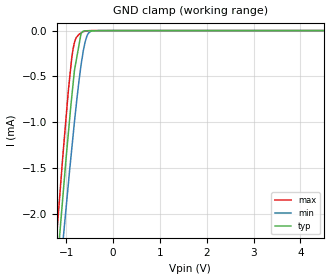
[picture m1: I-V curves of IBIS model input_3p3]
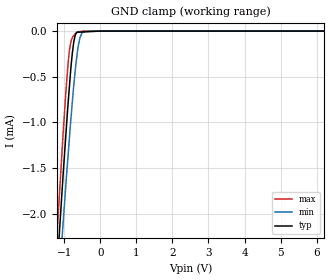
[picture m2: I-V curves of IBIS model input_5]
|Texas Instruments Incorporated
|Low-Power Rail-To-Rail Output 12-Bit Serial Input DAC
| Marketing part#   Digital Voltage Range   Package-type   #pins
| DAC7512E/250   2.7V - 5.5V   MSOP   8
| DAC7512E/250G4   2.7V - 5.5V   MSOP   8
| DAC7512E/2K5   2.7V - 5.5V   MSOP   8
| DAC7512E/2K5G4   2.7V - 5.5V   MSOP   8
[IBIS Ver]   3.2
[File name]   dac7512.ibs
[File Rev]   1.0
[Date]   7/6/2012
[Source]
| Texas Instruments Incorporated.
| Analog-eLab Design Center, HPA
| 12500 TI Blvd
| Dallas, TX -75243
| e-mail: elab_scm_ibis@list.ti.com
[Notes]   Revision History:
| Rev 1.0: 7/6/2012
| - Initial version of the model
| - Model generated from simulations in TISPICE
| - Model matched to SPICE simulation
| - C_comp although listed in numerical order of value are
|   obtained from varying PVT conditions. For PVT conditions for
|   each specific value refer the buffer description under
|   respective [Model]. IBIS model user is responsible for using
|   appropriate C_comp to simulate for Signal Integrity.
| - Model names with a trailing _3p3 contains the model for
|   3.3V [3.0V and 3.6V]. Model names with a trailing _5 contains
|   the model for 5.0V [4.5V and 5.5V].
[Disclaimer]
| This model is designed as an aid for customers of Texas Instruments.
| TI and its licensors and suppliers make no warranties, either expressed
| or implied, with respect to this  model, including the warranties of
| merchantability or fitness for a particular purpose. The model is
| provided solely on an "as is" basis. The entire risk as to its quality
| and performance is with the customer.
[Copyright]
(C) Copyright 2012 Texas Instruments Incorporated.All rights reserved.
|   DAC7512DGK
[Component]   DAC7512DGK
[Manufacturer]   TI
[Package]   |8 MSOP   -  DGK package
|   typ   min   max
R_pkg   0.0631   0.03789   0.07234
L_pkg   1.99460nH   1.78333nH   2.07644nH
C_pkg   0.41172pF   0.38717pF   0.42444pF
[Pin]  signal_name   model_name   R_pin   L_pin   C_pin
1   VDD   POWER   0.03793   1.74606nH  0.41528pF
2   NC   NC   0.00589   1.01766nH  0.34952pF
3   NC   NC   0.00589   1.01765nH  0.34952pF
4   VOUT   TERM   0.03789   1.78333nH  0.41083pF
5   _SYNC   INPUT   0.06966   2.04248nH  0.38717pF
6   SCLK   INPUT   0.07234   2.07644nH  0.42444pF
7   DIN   INPUT   0.07232   2.07614nH  0.42444pF
8   GND   GND   0.06967   2.04266nH  0.38717pF
|   Model Selectors
[Model Selector] INPUT
input_3p3   3.3V  digital input
input_5   5.0V  digital input
[Model Selector] TERM
term_3-3V  3.3V  nominal termination
term_5V   5.0V  nominal termination
[Model] term_3-3V
Model_type Terminator
C_comp   1.0e-20F  1.0e-20F  1.0e-20F
|   typ   min   max
[Voltage Range]   3.3V   3.0V   3.6V
[POWER Clamp Reference]   3.3V   3.0V   3.6V
[GND Clamp Reference]   0V   0V   0V
|Ambient Temperature   25   105   -40
|Junction Temperature
[Temperature Range]   25   105   -40
[Model] term_5V
Model_type Terminator
C_comp   1.0e-20F  1.0e-20F  1.0e-20F
|   typ   min   max
[Voltage Range]   5.0V   4.5V   5.5V
[POWER Clamp Reference]   5.0V   4.5V   5.5V
[GND Clamp Reference]   0V   0V   0V
|Ambient Temperature   25   105   -40
|Junction Temperature
[Temperature Range]   25   105   -40
| Models and submodels in the file (4): input_3p3 (Input), input_5 (Input), term_3-3V (Terminator), term_5V (Terminator)
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|   input_3p3 Model
[Model]   input_3p3
Model_type   Input
Vinl = 0.6
Vinh = 2.1
|   typ   min   max
|   (nom PVT)   (fast PVT)   (slow PVT)
|C_comp from frequency sweep method (F=30MHz)
|Average
|C_comp   3.437e-13   3.130e-13   3.752e-13
|C_comp from LC tank measurement(L=1nH)
|Average
|Resonant Frequency(Hz)   8.610e+09   8.850e+09   8.320e+09
C_comp   3.420e-13   3.237e-13   3.663e-13
| Where nom  PVT is Nominal Process, 3.3V, 25C
|   Fast PVT is Strong Process,  3.6V, -40C
|   Slow PVT is Weak Process,   3V, 105C
[Voltage Range]   3.3   3   3.6
|Ambient Temperature   25   105   -40
|Junction Temperature
[Temperature Range]   25   105   -40
[Power Clamp Reference]   3.3   3   3.6
[GND Clamp Reference]   0   0   0
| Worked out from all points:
|   GND clamp passes 1 mA (typ) near -0.93 V on its own axis
[GND Clamp]
|   Voltage   I(typ)   I(min)   I(max)
-3.3V     -16.02mA   -15.29mA   -16.79mA
-1.23V    -2.78mA    -3.213mA   -2.401mA
-1.072V   -1.809mA   -2.31mA    -1.36mA
-1.059V   -1.732mA   -2.238mA   -1.283mA
-956.4mV  -1.127mA   -1.679mA   -662.4uA
-880.8mV  -713.9uA   -1.282mA   -291.7uA
-825mV    -434.9uA   -994.8uA   -129.7uA
-683.1mV  -28.79uA   -372.9uA   -26.39uA
-650.1mV  -10.13uA   -265.1uA   -16.04uA
-525mV    -2.279uA   -27.09uA   -653.7nA
-327mV    -1.414uA   0A         0A
6.6V      0A         0A         0A
[POWER Clamp]
|   Voltage   I(typ)   I(min)   I(max)
-3.3V     0A         0A         0A
0V        0A         0A         0A
6.6V      0A         0A         0A
|   input_5 Model
[Model]   input_5
Model_type   Input
Vinl = 0.8
Vinh = 2.4
|   typ   min   max
|   (nom PVT)   (fast PVT)   (slow PVT)
|C_comp from frequency sweep method (F=30MHz)
|Average
|C_comp   3.176e-13   2.890e-13   3.459e-13
|C_comp from LC tank measurement(L=1nH)
|Average
|Resonant Frequency(Hz)   8.610e+09   8.850e+09   8.320e+09
C_comp   3.420e-13   3.237e-13   3.663e-13
| Where nom  PVT is Nominal Process, 5V, 25C
|   Fast PVT is Strong Process,  5.5V, -40C
|   Slow PVT is Weak Process,   4.5V, 105C
[Voltage Range]   5   4.5   5.5
|Ambient Temperature   25   105   -40
|Junction Temperature
[Temperature Range]   25   105   -40
[Power Clamp Reference]   5   4.5   5.5
[GND Clamp Reference]   0   0   0
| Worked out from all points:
|   GND clamp passes 1 mA (typ) near -0.94 V on its own axis
[GND Clamp]
|   Voltage   I(typ)   I(min)   I(max)
-5V       -26.98mA   -25.29mA   -28.67mA
-1.247V   -2.865mA   -3.292mA   -2.503mA
-1.04V    -1.599mA   -2.124mA   -1.151mA
-957.5mV  -1.125mA   -1.675mA   -658uA
-858.5mV  -595.5uA   -1.159mA   -205.9uA
-810mV    -360.5uA   -918.3uA   -103.1uA
-740mV    -118.6uA   -593.7uA   -48.6uA
-660mV    -12.99uA   -294.2uA   -18.37uA
-572mV    -11.25uA   -76.33uA   -4.871uA
-509mV    -10.01uA   -16.83uA   -1.756uA
-369.5mV  -7.27uA    0A         0A
10V       0A         0A         0A
[POWER Clamp]
|   Voltage   I(typ)   I(min)   I(max)
-5V       0A         0A         0A
0V        0A         0A         0A
10V       0A         0A         0A
